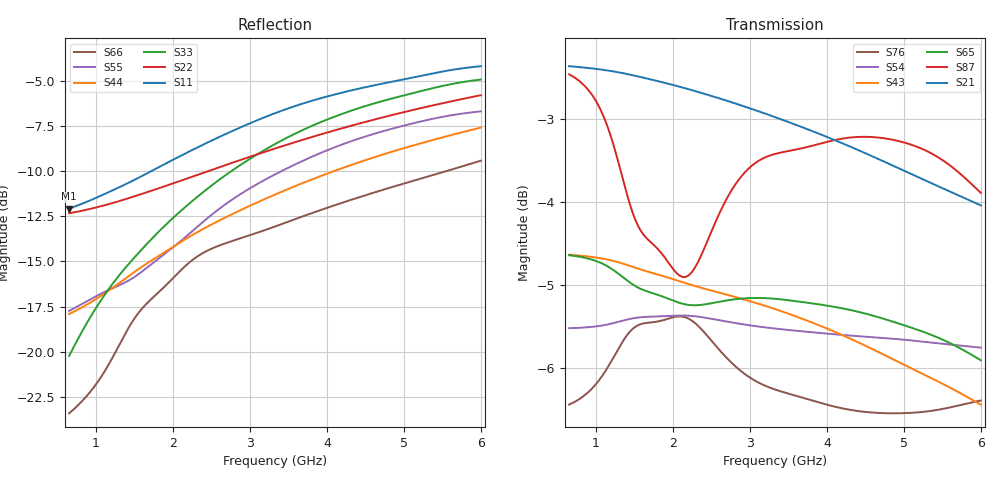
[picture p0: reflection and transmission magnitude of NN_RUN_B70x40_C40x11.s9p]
! IGNION VIRTUAL ANTENNA LIBRARY
! NN_RUN_B70x40_C40x11
! Virtual Antenna™ RUN mXTEND™: NN02-224 12.0 mm x 3.0 mm x 2.4 mm
! https://ignion.io/product/run-mxtend/
! Board: 70 mm x 40 mm
! Clearance Area: 40 mm x 11 mm
! Feeding line: L-shape; 11mm x 2mm and 5mm x 2mm
! Applications: Fleet management, IoT
! Frequency range 0.65GHz to 6GHz, step 10MHz
! Number of ports 9
! This product and its use is protected by at least one or more of the following patents and patent
! applications US 8,203,492 B2; US 8,237,615 B2; PCT/EP2013/064692; WO 2014/012842 A1; US 2019/190122 A1;
! US 62/072,671; and other domestic and international patents pending. Additional information about
! patents related to this product is available at https://ignion.io/files/Patent-list-NN.pdf, all
! rights reserved. Copyright, Ignion 2021.
! Need more help? Your platform is much different than these examples in the manual? Use our
! Fast Track service (https://ignion.io/fast-track/), for free, and get a personalized antenna design in
! just 24 hours.
! Touchstone port 1 = "Series Port"
! Touchstone port 2 = "Shunt Port"
! Touchstone port 3 = "Series Port"
! Touchstone port 4 = "Shunt Port"
! Touchstone port 5 = "Series Port"
! Touchstone port 6 = "Shunt Port"
! Touchstone port 7 = "Series Port"
! Touchstone port 8 = "Shunt Port"
! Touchstone port 9 = "Series Port"
! IE3D S-Parameters Output Version 2.0
# GHZ S MA R 50
! Nport = 9
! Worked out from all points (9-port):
!   536 points, 650 MHz to 6 GHz, reference 50 ohm
!   strongest paths, dB at 650 MHz, 1.99 GHz, 3.33 GHz, 4.67 GHz, 6 GHz:
!     S21: -2.4, -2.6, -3.0, -3.5, -4.0
!     S87: -2.5, -4.8, -3.4, -3.2, -3.9
!     S65: -4.6, -5.2, -5.2, -5.4, -5.9
!     S43: -4.6, -4.9, -5.3, -5.8, -6.4
!     S54: -5.5, -5.4, -5.5, -5.6, -5.8
!     S76: -6.4, -5.4, -6.3, -6.5, -6.4
!   lowest |S11| = -12.1 dB at 650 MHz (marker M1), VSWR 1.66, Z = 31.1 + j7.45 ohm
!   |S11| at or under -10 dB: start of sweep to 1.721 GHz
